(* Logix 5000 AddOnInstructionDefinition export Banner_LTF_Param_v4; software revision 33.00; part 2 of 3 *)
(* tags used below, declared in another part *)
   LTF : Banner_LTF_v4;
   Port_Data : Banner_IOL_Port_v4;
   Port : DINT;
   Local_Control : DINT;
   Command_Being_Processed : BOOL;
   Update_Archive : BOOL;
   Index_Write_Control : DINT;
   Index_Write_Inprocess : INT;
   Inprocess_Index : DINT;
(* Banner_LTF_Param_v4, continued *)

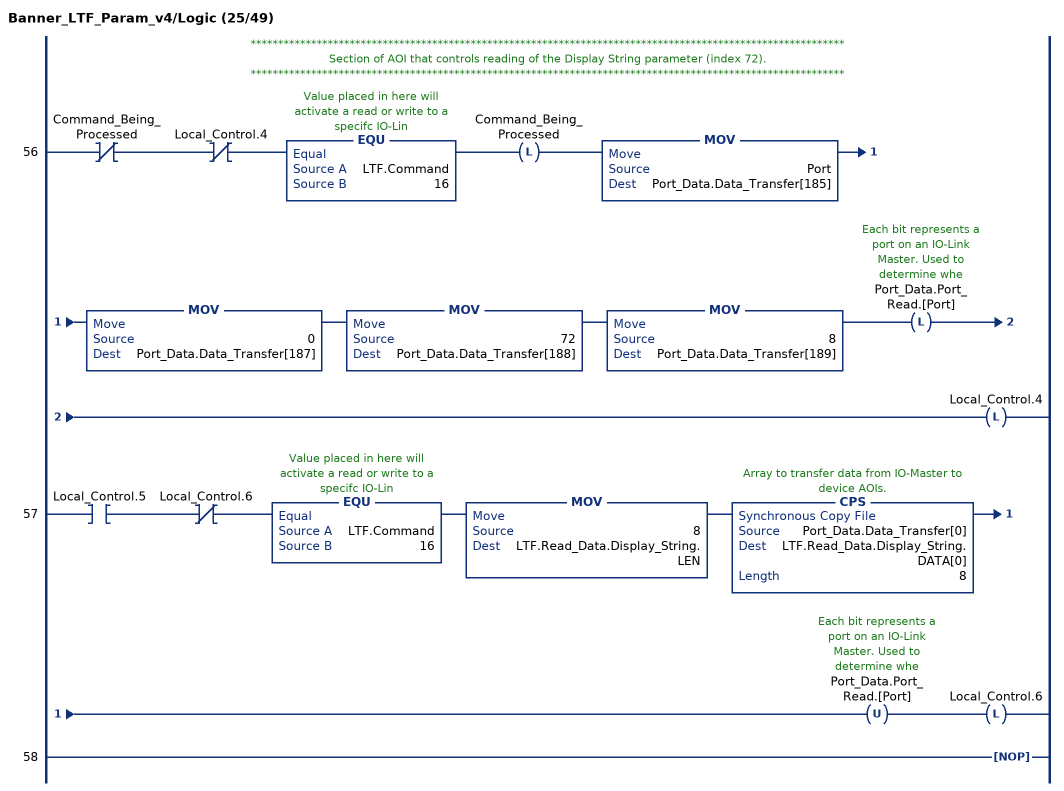
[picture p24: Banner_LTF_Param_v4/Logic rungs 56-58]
   // ************************************************************************************************************
   // Section of AOI that controls reading of the Display String parameter (index 72).
   // ************************************************************************************************************
   56: XIO(Command_Being_Processed)XIO(Local_Control.4)EQU(LTF.Command,16)OTL(Command_Being_Processed)MOV(Port,Port_Data.Data_Transfer[185])MOV(0,Port_Data.Data_Transfer[187])MOV(72,Port_Data.Data_Transfer[188])MOV(8,Port_Data.Data_Transfer[189])OTL(Port_Data.Port_Read.[Port])OTL(Local_Control.4);
   57: XIC(Local_Control.5)XIO(Local_Control.6)EQU(LTF.Command,16)MOV(8,LTF.Read_Data.Display_String.LEN)CPS(Port_Data.Data_Transfer[0],LTF.Read_Data.Display_String.DATA[0],8)OTU(Port_Data.Port_Read.[Port])OTL(Local_Control.6);
   58: NOP();
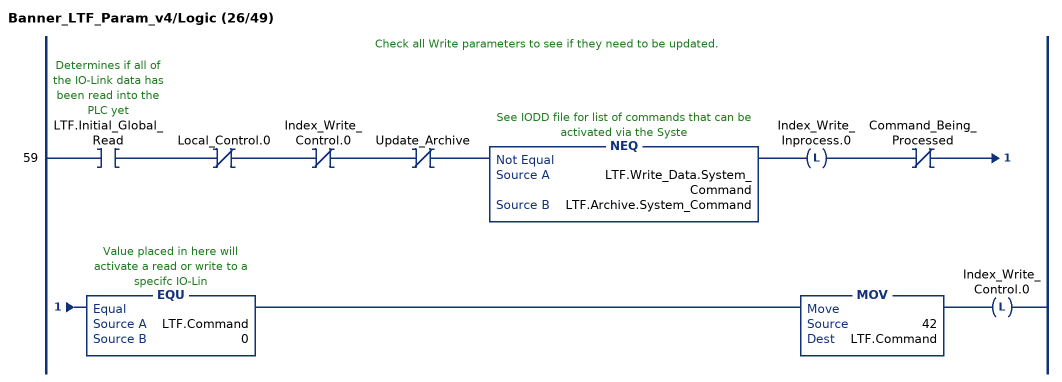
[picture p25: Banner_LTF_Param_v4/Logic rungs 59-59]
   // Check all Write parameters to see if they need to be updated.
   59: XIC(LTF.Initial_Global_Read)XIO(Local_Control.0)XIO(Index_Write_Control.0)XIO(Update_Archive)NEQ(LTF.Write_Data.System_Command,LTF.Archive.System_Command)OTL(Index_Write_Inprocess.0)XIO(Command_Being_Processed)EQU(LTF.Command,0)MOV(42,LTF.Command)OTL(Index_Write_Control.0);
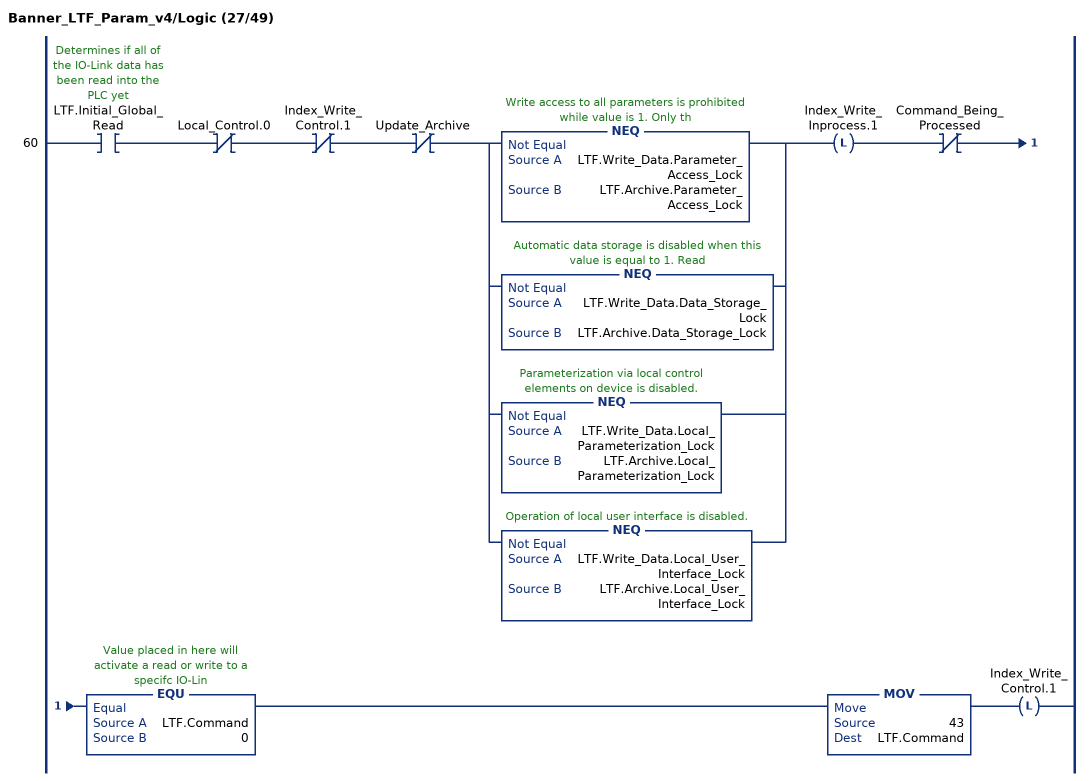
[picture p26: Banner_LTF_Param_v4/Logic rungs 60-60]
   60: XIC(LTF.Initial_Global_Read)XIO(Local_Control.0)XIO(Index_Write_Control.1)XIO(Update_Archive)[NEQ(LTF.Write_Data.Parameter_Access_Lock,LTF.Archive.Parameter_Access_Lock) ,NEQ(LTF.Write_Data.Data_Storage_Lock,LTF.Archive.Data_Storage_Lock) ,NEQ(LTF.Write_Data.Local_Parameterization_Lock,LTF.Archive.Local_Parameterization_Lock) ,NEQ(LTF.Write_Data.Local_User_Interface_Lock,LTF.Archive.Local_User_Interface_Lock) ]OTL(Index_Write_Inprocess.1)XIO(Command_Being_Processed)EQU(LTF.Command,0)MOV(43,LTF.Command)OTL(Index_Write_Control.1);
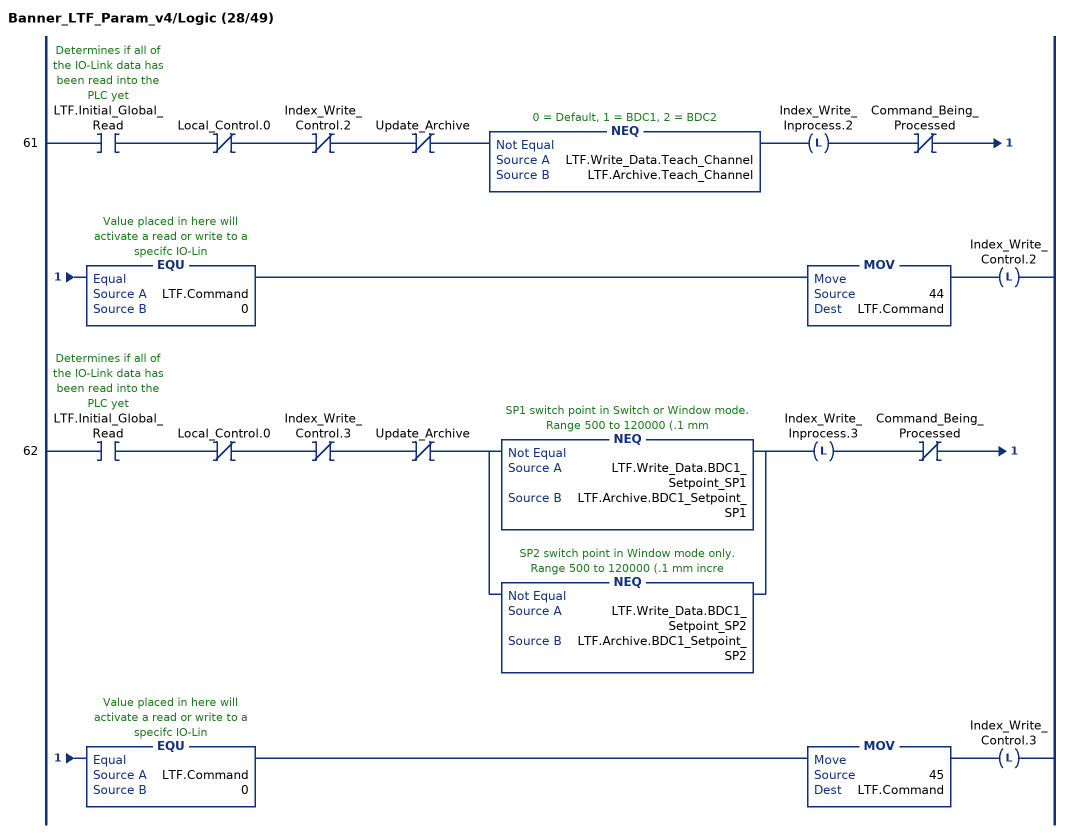
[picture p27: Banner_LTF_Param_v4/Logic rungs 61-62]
   61: XIC(LTF.Initial_Global_Read)XIO(Local_Control.0)XIO(Index_Write_Control.2)XIO(Update_Archive)NEQ(LTF.Write_Data.Teach_Channel,LTF.Archive.Teach_Channel)OTL(Index_Write_Inprocess.2)XIO(Command_Being_Processed)EQU(LTF.Command,0)MOV(44,LTF.Command)OTL(Index_Write_Control.2);
   62: XIC(LTF.Initial_Global_Read)XIO(Local_Control.0)XIO(Index_Write_Control.3)XIO(Update_Archive)[NEQ(LTF.Write_Data.BDC1_Setpoint_SP1,LTF.Archive.BDC1_Setpoint_SP1) ,NEQ(LTF.Write_Data.BDC1_Setpoint_SP2,LTF.Archive.BDC1_Setpoint_SP2) ]OTL(Index_Write_Inprocess.3)XIO(Command_Being_Processed)EQU(LTF.Command,0)MOV(45,LTF.Command)OTL(Index_Write_Control.3);
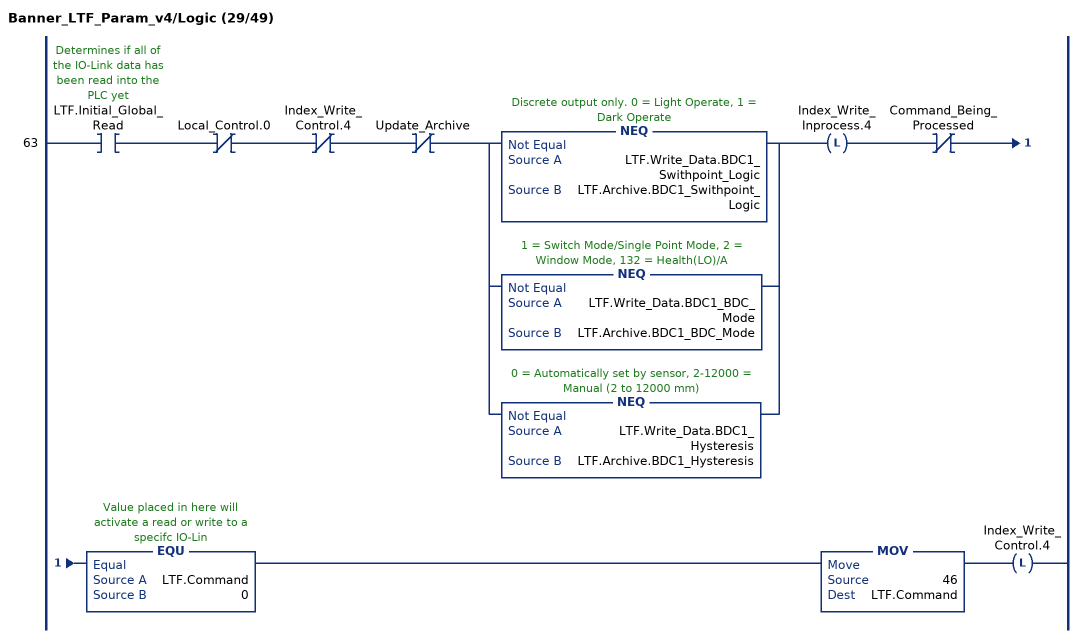
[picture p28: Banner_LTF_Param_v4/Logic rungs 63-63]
   63: XIC(LTF.Initial_Global_Read)XIO(Local_Control.0)XIO(Index_Write_Control.4)XIO(Update_Archive)[NEQ(LTF.Write_Data.BDC1_Swithpoint_Logic,LTF.Archive.BDC1_Swithpoint_Logic) ,NEQ(LTF.Write_Data.BDC1_BDC_Mode,LTF.Archive.BDC1_BDC_Mode) ,NEQ(LTF.Write_Data.BDC1_Hysteresis,LTF.Archive.BDC1_Hysteresis) ]OTL(Index_Write_Inprocess.4)XIO(Command_Being_Processed)EQU(LTF.Command,0)MOV(46,LTF.Command)OTL(Index_Write_Control.4);
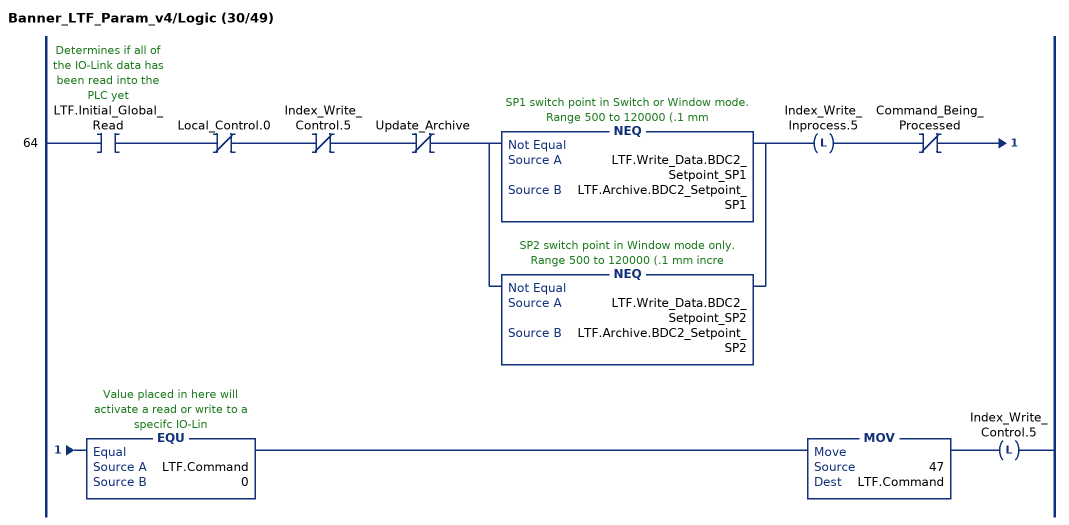
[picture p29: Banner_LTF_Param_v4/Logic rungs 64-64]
   64: XIC(LTF.Initial_Global_Read)XIO(Local_Control.0)XIO(Index_Write_Control.5)XIO(Update_Archive)[NEQ(LTF.Write_Data.BDC2_Setpoint_SP1,LTF.Archive.BDC2_Setpoint_SP1) ,NEQ(LTF.Write_Data.BDC2_Setpoint_SP2,LTF.Archive.BDC2_Setpoint_SP2) ]OTL(Index_Write_Inprocess.5)XIO(Command_Being_Processed)EQU(LTF.Command,0)MOV(47,LTF.Command)OTL(Index_Write_Control.5);
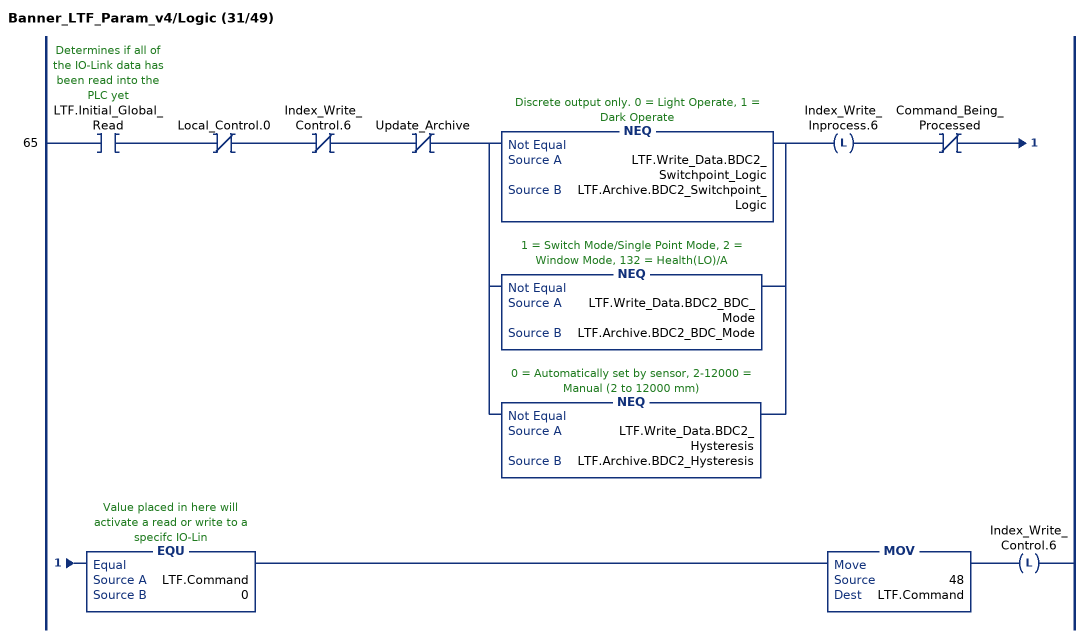
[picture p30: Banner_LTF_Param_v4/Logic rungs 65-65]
   65: XIC(LTF.Initial_Global_Read)XIO(Local_Control.0)XIO(Index_Write_Control.6)XIO(Update_Archive)[NEQ(LTF.Write_Data.BDC2_Switchpoint_Logic,LTF.Archive.BDC2_Switchpoint_Logic) ,NEQ(LTF.Write_Data.BDC2_BDC_Mode,LTF.Archive.BDC2_BDC_Mode) ,NEQ(LTF.Write_Data.BDC2_Hysteresis,LTF.Archive.BDC2_Hysteresis) ]OTL(Index_Write_Inprocess.6)XIO(Command_Being_Processed)EQU(LTF.Command,0)MOV(48,LTF.Command)OTL(Index_Write_Control.6);
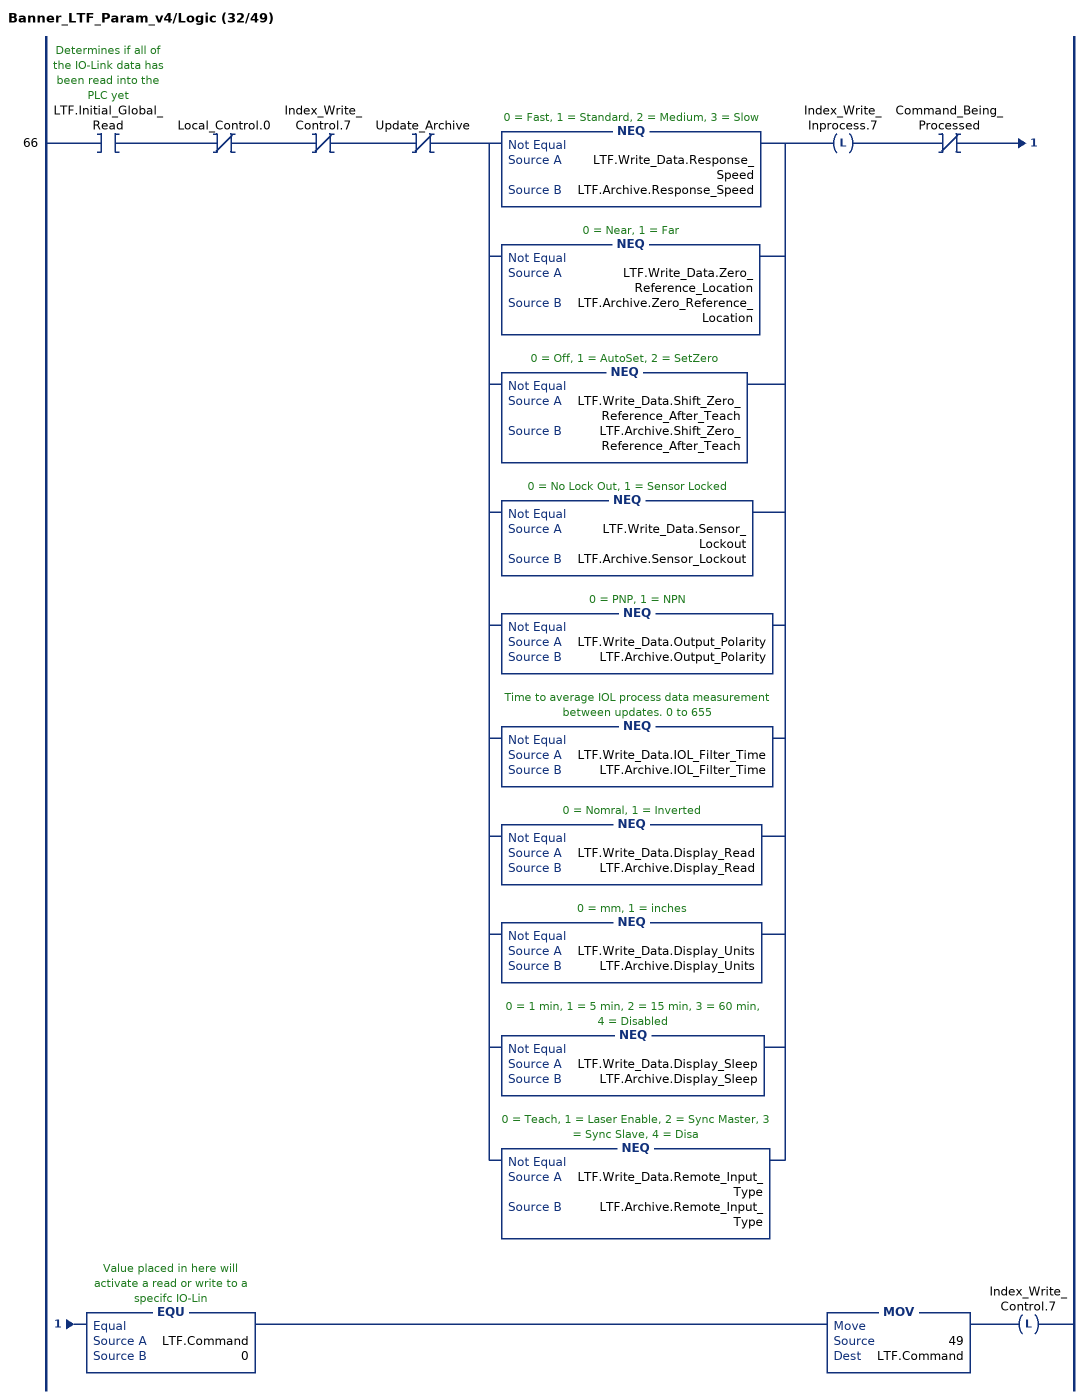
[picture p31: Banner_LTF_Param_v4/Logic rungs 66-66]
   66: XIC(LTF.Initial_Global_Read)XIO(Local_Control.0)XIO(Index_Write_Control.7)XIO(Update_Archive)[NEQ(LTF.Write_Data.Response_Speed,LTF.Archive.Response_Speed) ,NEQ(LTF.Write_Data.Zero_Reference_Location,LTF.Archive.Zero_Reference_Location) ,NEQ(LTF.Write_Data.Shift_Zero_Reference_After_Teach,LTF.Archive.Shift_Zero_Reference_After_Teach) ,NEQ(LTF.Write_Data.Sensor_Lockout,LTF.Archive.Sensor_Lockout) ,NEQ(LTF.Write_Data.Output_Polarity,LTF.Archive.Output_Polarity) ,NEQ(LTF.Write_Data.IOL_Filter_Time,LTF.Archive.IOL_Filter_Time) ,NEQ(LTF.Write_Data.Display_Read,LTF.Archive.Display_Read) ,NEQ(LTF.Write_Data.Display_Units,LTF.Archive.Display_Units) ,NEQ(LTF.Write_Data.Display_Sleep,LTF.Archive.Display_Sleep) ,NEQ(LTF.Write_Data.Remote_Input_Type,LTF.Archive.Remote_Input_Type) ]OTL(Index_Write_Inprocess.7)XIO(Command_Being_Processed)EQU(LTF.Command,0)MOV(49,LTF.Command)OTL(Index_Write_Control.7);
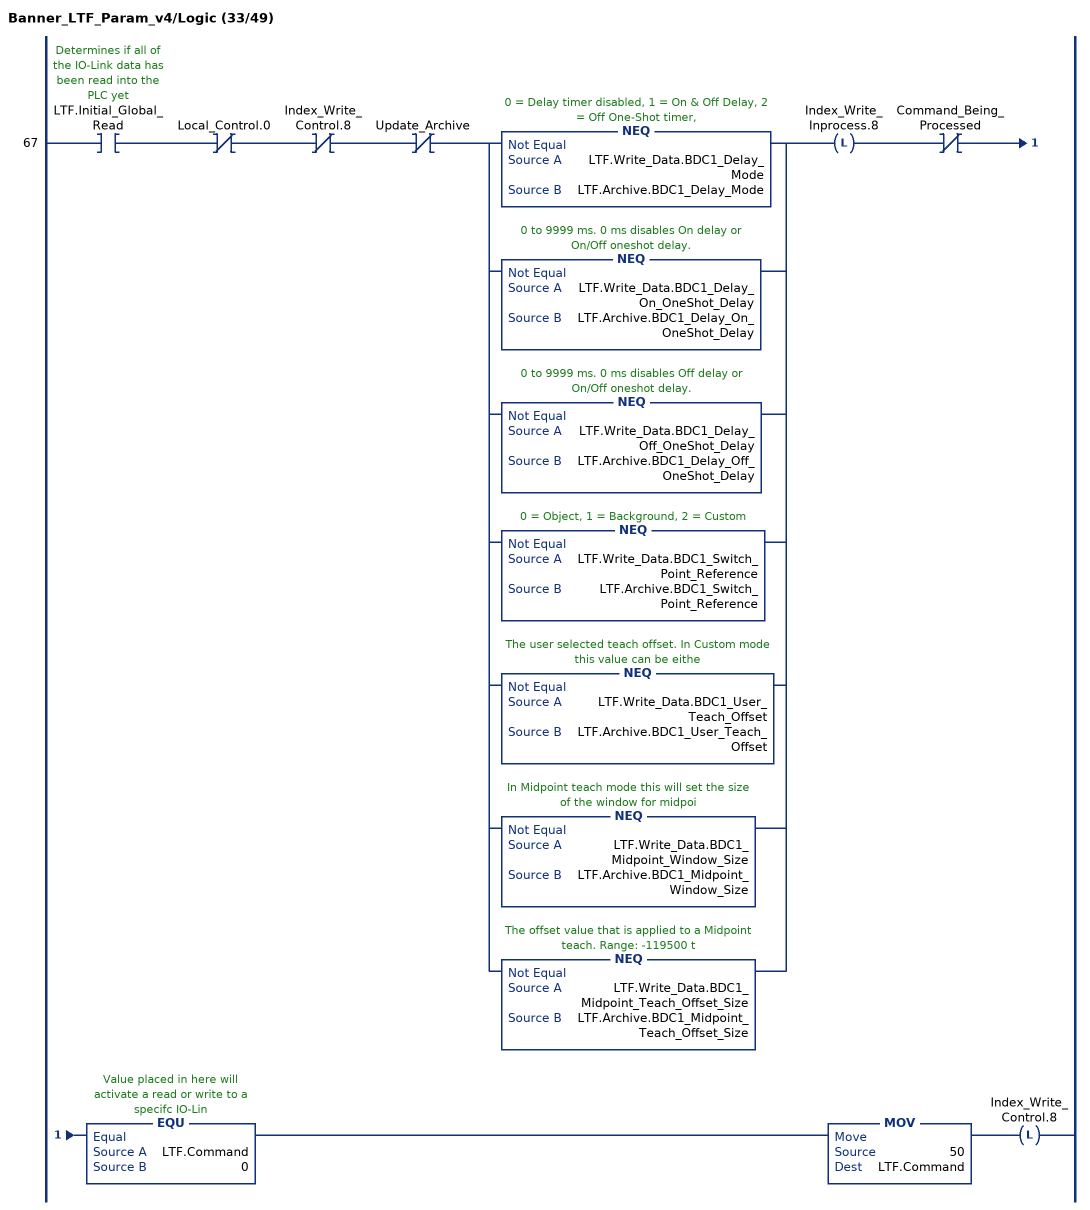
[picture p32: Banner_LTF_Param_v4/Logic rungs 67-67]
   67: XIC(LTF.Initial_Global_Read)XIO(Local_Control.0)XIO(Index_Write_Control.8)XIO(Update_Archive)[NEQ(LTF.Write_Data.BDC1_Delay_Mode,LTF.Archive.BDC1_Delay_Mode) ,NEQ(LTF.Write_Data.BDC1_Delay_On_OneShot_Delay,LTF.Archive.BDC1_Delay_On_OneShot_Delay) ,NEQ(LTF.Write_Data.BDC1_Delay_Off_OneShot_Delay,LTF.Archive.BDC1_Delay_Off_OneShot_Delay) ,NEQ(LTF.Write_Data.BDC1_Switch_Point_Reference,LTF.Archive.BDC1_Switch_Point_Reference) ,NEQ(LTF.Write_Data.BDC1_User_Teach_Offset,LTF.Archive.BDC1_User_Teach_Offset) ,NEQ(LTF.Write_Data.BDC1_Midpoint_Window_Size,LTF.Archive.BDC1_Midpoint_Window_Size) ,NEQ(LTF.Write_Data.BDC1_Midpoint_Teach_Offset_Size,LTF.Archive.BDC1_Midpoint_Teach_Offset_Size) ]OTL(Index_Write_Inprocess.8)XIO(Command_Being_Processed)EQU(LTF.Command,0)MOV(50,LTF.Command)OTL(Index_Write_Control.8);
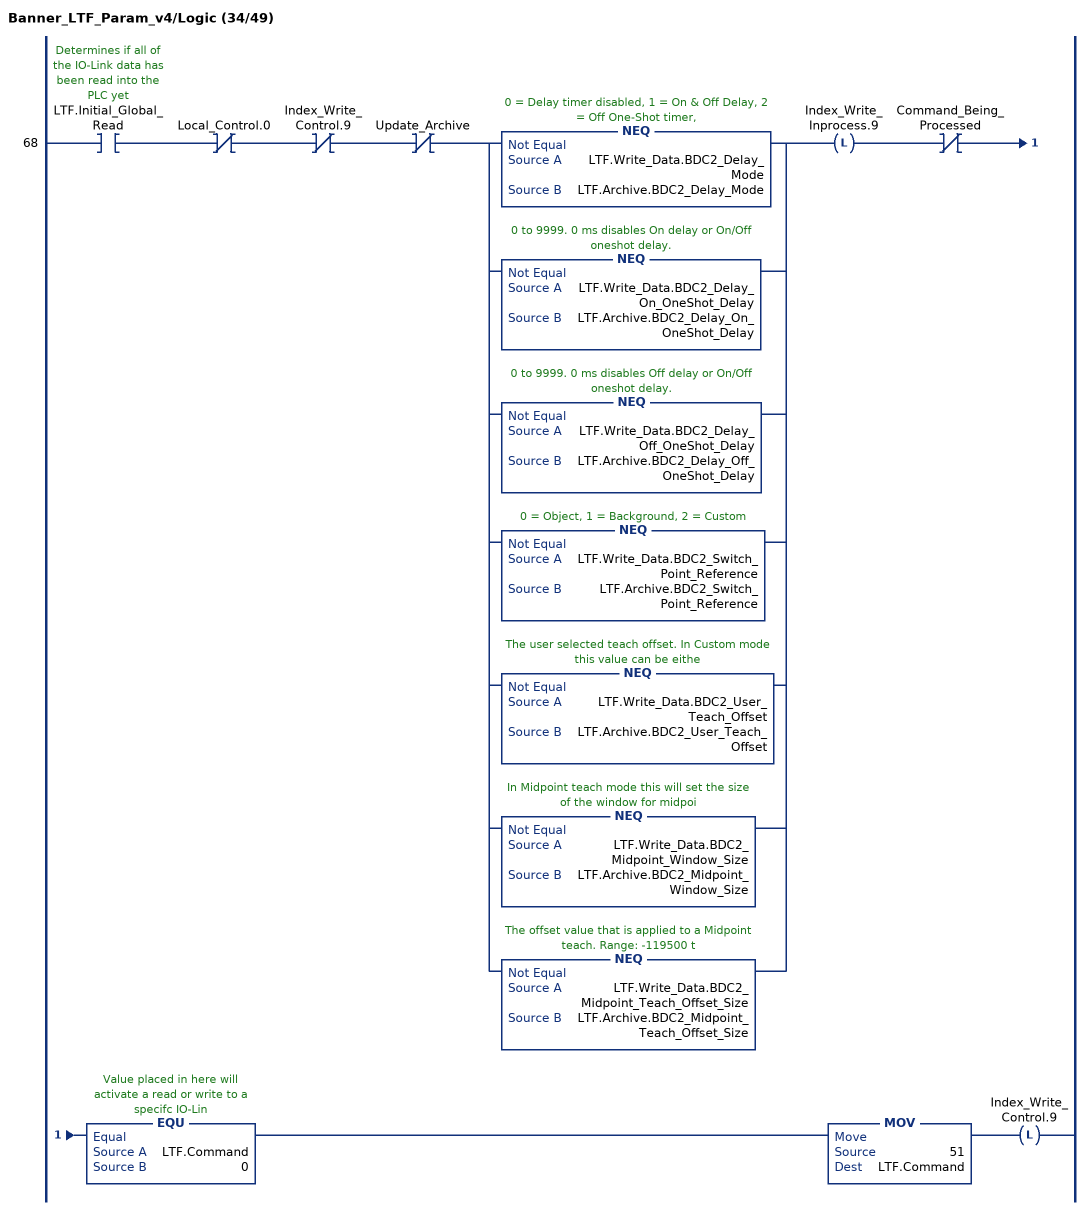
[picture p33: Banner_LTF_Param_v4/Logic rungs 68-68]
   68: XIC(LTF.Initial_Global_Read)XIO(Local_Control.0)XIO(Index_Write_Control.9)XIO(Update_Archive)[NEQ(LTF.Write_Data.BDC2_Delay_Mode,LTF.Archive.BDC2_Delay_Mode) ,NEQ(LTF.Write_Data.BDC2_Delay_On_OneShot_Delay,LTF.Archive.BDC2_Delay_On_OneShot_Delay) ,NEQ(LTF.Write_Data.BDC2_Delay_Off_OneShot_Delay,LTF.Archive.BDC2_Delay_Off_OneShot_Delay) ,NEQ(LTF.Write_Data.BDC2_Switch_Point_Reference,LTF.Archive.BDC2_Switch_Point_Reference) ,NEQ(LTF.Write_Data.BDC2_User_Teach_Offset,LTF.Archive.BDC2_User_Teach_Offset) ,NEQ(LTF.Write_Data.BDC2_Midpoint_Window_Size,LTF.Archive.BDC2_Midpoint_Window_Size) ,NEQ(LTF.Write_Data.BDC2_Midpoint_Teach_Offset_Size,LTF.Archive.BDC2_Midpoint_Teach_Offset_Size) ]OTL(Index_Write_Inprocess.9)XIO(Command_Being_Processed)EQU(LTF.Command,0)MOV(51,LTF.Command)OTL(Index_Write_Control.9);
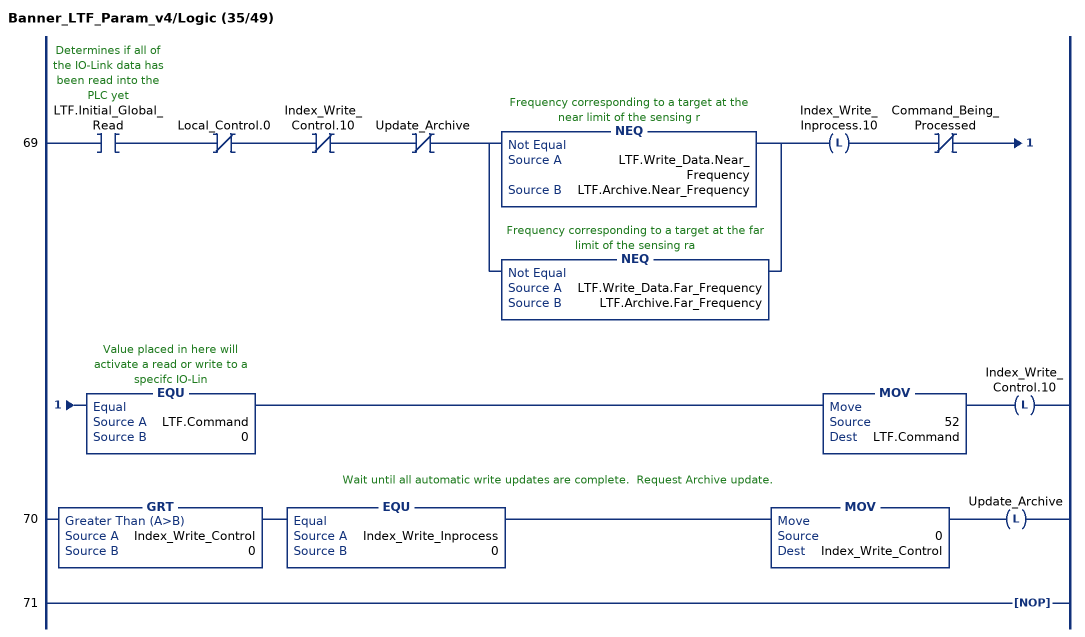
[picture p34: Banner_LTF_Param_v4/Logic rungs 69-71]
   69: XIC(LTF.Initial_Global_Read)XIO(Local_Control.0)XIO(Index_Write_Control.10)XIO(Update_Archive)[NEQ(LTF.Write_Data.Near_Frequency,LTF.Archive.Near_Frequency) ,NEQ(LTF.Write_Data.Far_Frequency,LTF.Archive.Far_Frequency) ]OTL(Index_Write_Inprocess.10)XIO(Command_Being_Processed)EQU(LTF.Command,0)MOV(52,LTF.Command)OTL(Index_Write_Control.10);
   // Wait until all automatic write updates are complete.  Request Archive update.
   70: GRT(Index_Write_Control,0)EQU(Index_Write_Inprocess,0)MOV(0,Index_Write_Control)OTL(Update_Archive);
   71: NOP();
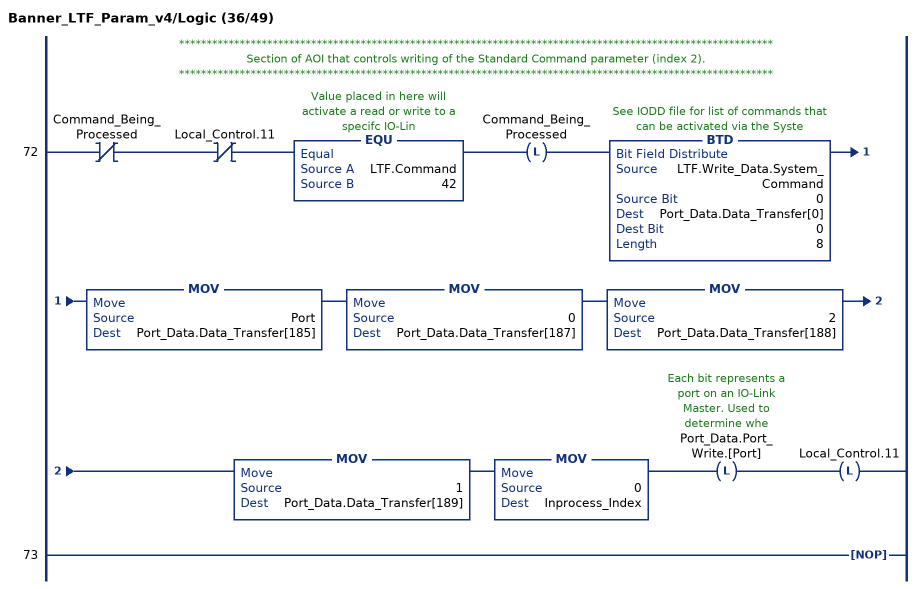
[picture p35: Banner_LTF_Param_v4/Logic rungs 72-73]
   // ************************************************************************************************************
   // Section of AOI that controls writing of the Standard Command parameter (index 2).
   // ************************************************************************************************************
   72: XIO(Command_Being_Processed)XIO(Local_Control.11)EQU(LTF.Command,42)OTL(Command_Being_Processed)BTD(LTF.Write_Data.System_Command,0,Port_Data.Data_Transfer[0],0,8)MOV(Port,Port_Data.Data_Transfer[185])MOV(0,Port_Data.Data_Transfer[187])MOV(2,Port_Data.Data_Transfer[188])MOV(1,Port_Data.Data_Transfer[189])MOV(0,Inprocess_Index)OTL(Port_Data.Port_Write.[Port])OTL(Local_Control.11);
   73: NOP();
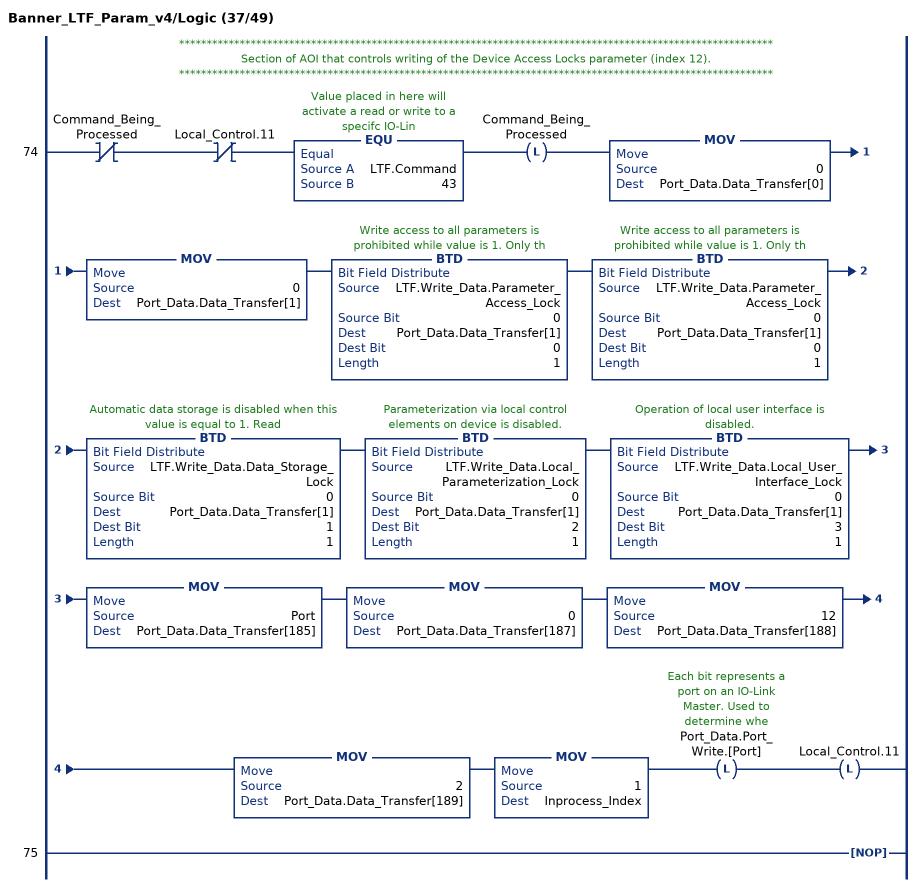
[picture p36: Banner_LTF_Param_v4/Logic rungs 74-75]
   // ************************************************************************************************************
   // Section of AOI that controls writing of the Device Access Locks parameter (index 12).
   // ************************************************************************************************************
   74: XIO(Command_Being_Processed)XIO(Local_Control.11)EQU(LTF.Command,43)OTL(Command_Being_Processed)MOV(0,Port_Data.Data_Transfer[0])MOV(0,Port_Data.Data_Transfer[1])BTD(LTF.Write_Data.Parameter_Access_Lock,0,Port_Data.Data_Transfer[1],0,1)BTD(LTF.Write_Data.Parameter_Access_Lock,0,Port_Data.Data_Transfer[1],0,1)BTD(LTF.Write_Data.Data_Storage_Lock,0,Port_Data.Data_Transfer[1],1,1)BTD(LTF.Write_Data.Local_Parameterization_Lock,0,Port_Data.Data_Transfer[1],2,1)BTD(LTF.Write_Data.Local_User_Interface_Lock,0,Port_Data.Data_Transfer[1],3,1)MOV(Port,Port_Data.Data_Transfer[185])MOV(0,Port_Data.Data_Transfer[187])MOV(12,Port_Data.Data_Transfer[188])MOV(2,Port_Data.Data_Transfer[189])MOV(1,Inprocess_Index)OTL(Port_Data.Port_Write.[Port])OTL(Local_Control.11);
   75: NOP();
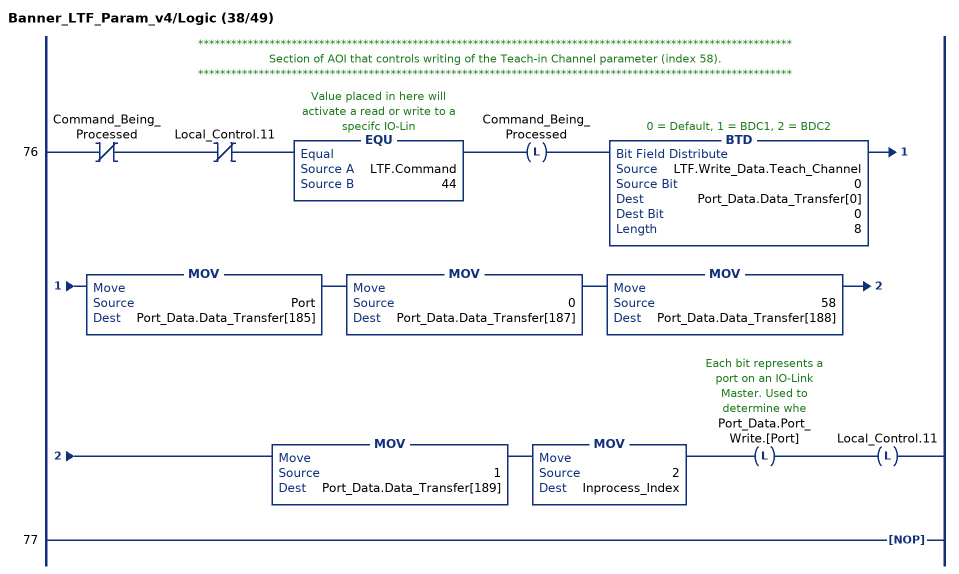
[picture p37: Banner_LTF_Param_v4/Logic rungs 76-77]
   // ************************************************************************************************************
   // Section of AOI that controls writing of the Teach-in Channel parameter (index 58).
   // ************************************************************************************************************
   76: XIO(Command_Being_Processed)XIO(Local_Control.11)EQU(LTF.Command,44)OTL(Command_Being_Processed)BTD(LTF.Write_Data.Teach_Channel,0,Port_Data.Data_Transfer[0],0,8)MOV(Port,Port_Data.Data_Transfer[185])MOV(0,Port_Data.Data_Transfer[187])MOV(58,Port_Data.Data_Transfer[188])MOV(1,Port_Data.Data_Transfer[189])MOV(2,Inprocess_Index)OTL(Port_Data.Port_Write.[Port])OTL(Local_Control.11);
   77: NOP();
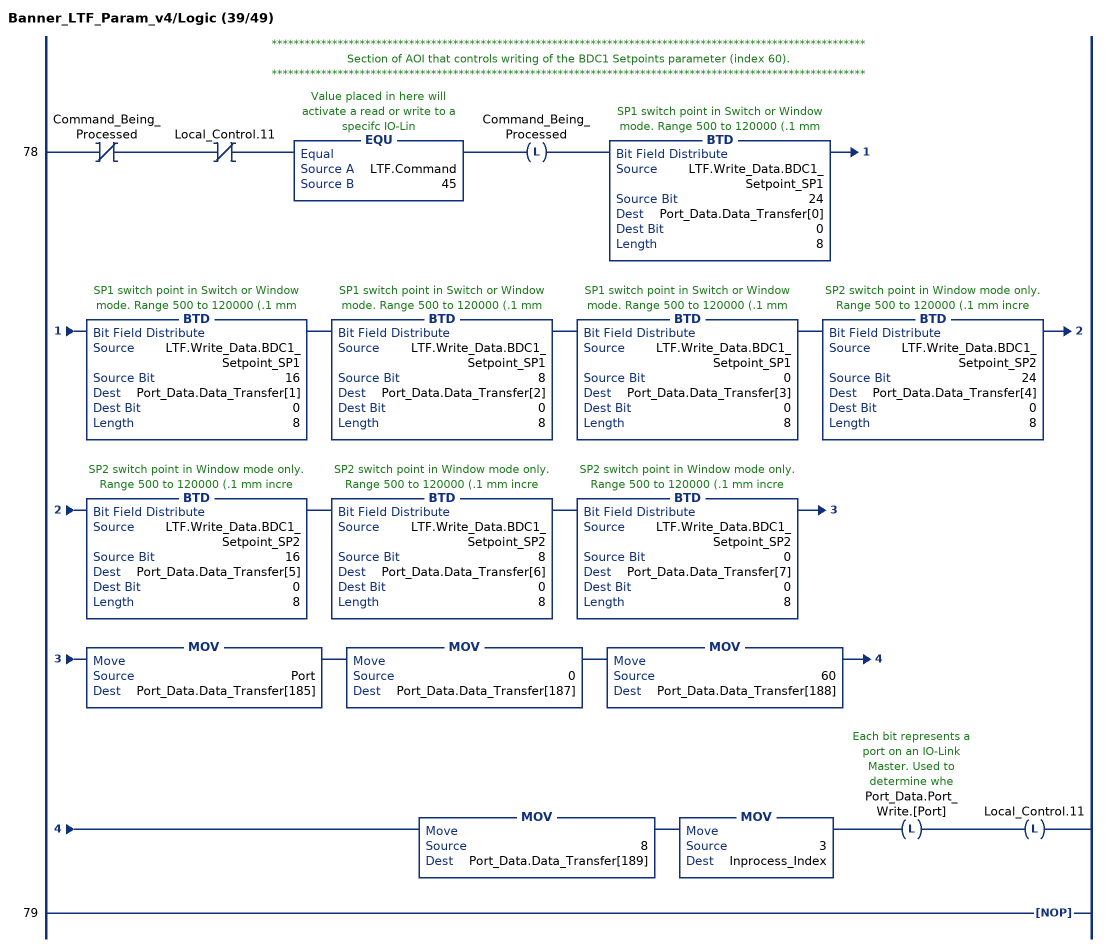
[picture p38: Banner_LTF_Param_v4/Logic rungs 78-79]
   // ************************************************************************************************************
   // Section of AOI that controls writing of the BDC1 Setpoints parameter (index 60).
   // ************************************************************************************************************
   78: XIO(Command_Being_Processed)XIO(Local_Control.11)EQU(LTF.Command,45)OTL(Command_Being_Processed)BTD(LTF.Write_Data.BDC1_Setpoint_SP1,24,Port_Data.Data_Transfer[0],0,8)BTD(LTF.Write_Data.BDC1_Setpoint_SP1,16,Port_Data.Data_Transfer[1],0,8)BTD(LTF.Write_Data.BDC1_Setpoint_SP1,8,Port_Data.Data_Transfer[2],0,8)BTD(LTF.Write_Data.BDC1_Setpoint_SP1,0,Port_Data.Data_Transfer[3],0,8)BTD(LTF.Write_Data.BDC1_Setpoint_SP2,24,Port_Data.Data_Transfer[4],0,8)BTD(LTF.Write_Data.BDC1_Setpoint_SP2,16,Port_Data.Data_Transfer[5],0,8)BTD(LTF.Write_Data.BDC1_Setpoint_SP2,8,Port_Data.Data_Transfer[6],0,8)BTD(LTF.Write_Data.BDC1_Setpoint_SP2,0,Port_Data.Data_Transfer[7],0,8)MOV(Port,Port_Data.Data_Transfer[185])MOV(0,Port_Data.Data_Transfer[187])MOV(60,Port_Data.Data_Transfer[188])MOV(8,Port_Data.Data_Transfer[189])MOV(3,Inprocess_Index)OTL(Port_Data.Port_Write.[Port])OTL(Local_Control.11);
   79: NOP();
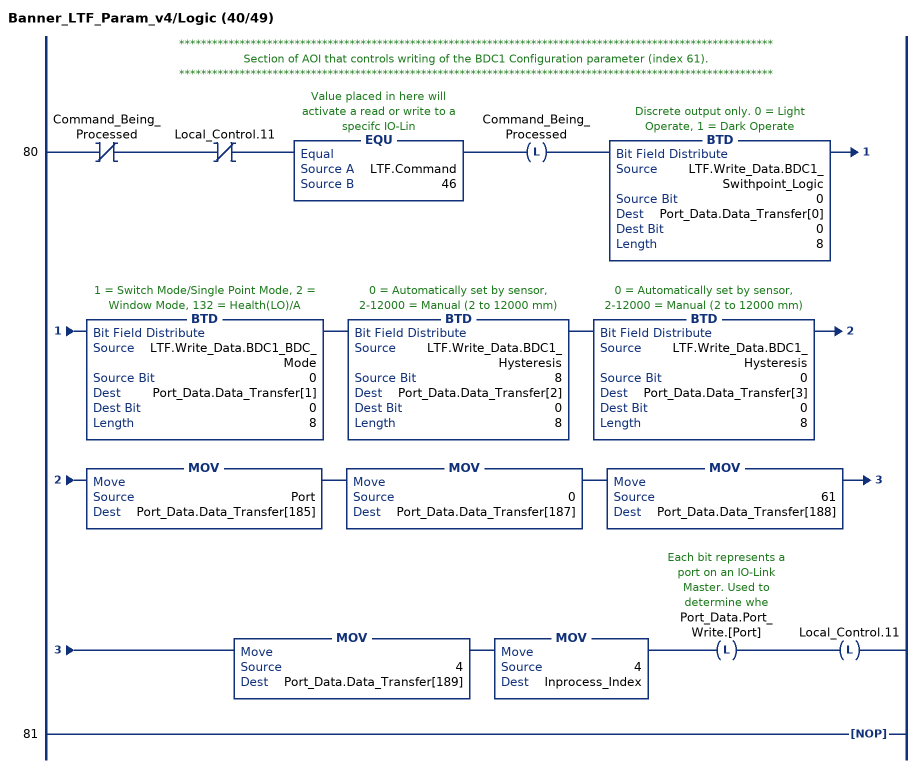
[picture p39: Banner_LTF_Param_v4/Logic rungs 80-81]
   // ************************************************************************************************************
   // Section of AOI that controls writing of the BDC1 Configuration parameter (index 61).
   // ************************************************************************************************************
   80: XIO(Command_Being_Processed)XIO(Local_Control.11)EQU(LTF.Command,46)OTL(Command_Being_Processed)BTD(LTF.Write_Data.BDC1_Swithpoint_Logic,0,Port_Data.Data_Transfer[0],0,8)BTD(LTF.Write_Data.BDC1_BDC_Mode,0,Port_Data.Data_Transfer[1],0,8)BTD(LTF.Write_Data.BDC1_Hysteresis,8,Port_Data.Data_Transfer[2],0,8)BTD(LTF.Write_Data.BDC1_Hysteresis,0,Port_Data.Data_Transfer[3],0,8)MOV(Port,Port_Data.Data_Transfer[185])MOV(0,Port_Data.Data_Transfer[187])MOV(61,Port_Data.Data_Transfer[188])MOV(4,Port_Data.Data_Transfer[189])MOV(4,Inprocess_Index)OTL(Port_Data.Port_Write.[Port])OTL(Local_Control.11);
   81: NOP();
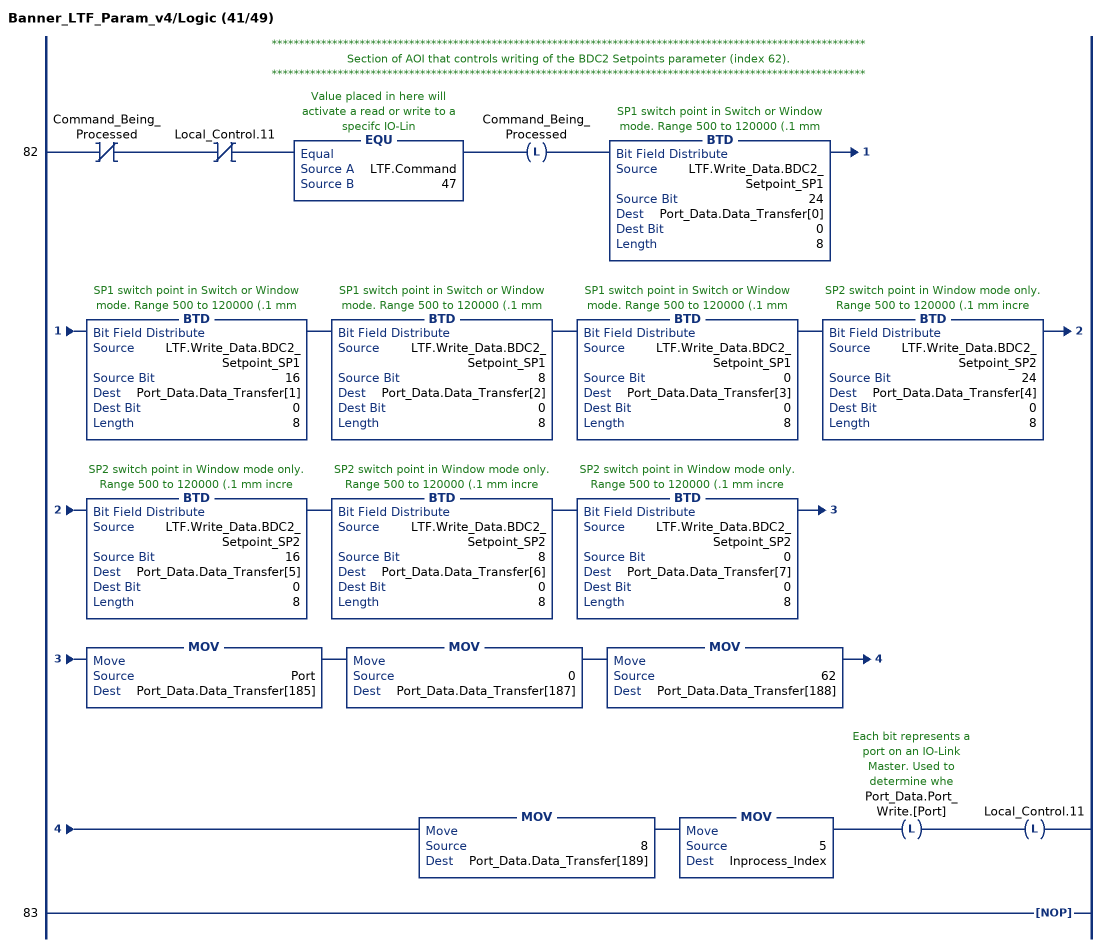
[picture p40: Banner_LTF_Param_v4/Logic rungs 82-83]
   // ************************************************************************************************************
   // Section of AOI that controls writing of the BDC2 Setpoints parameter (index 62).
   // ************************************************************************************************************
   82: XIO(Command_Being_Processed)XIO(Local_Control.11)EQU(LTF.Command,47)OTL(Command_Being_Processed)BTD(LTF.Write_Data.BDC2_Setpoint_SP1,24,Port_Data.Data_Transfer[0],0,8)BTD(LTF.Write_Data.BDC2_Setpoint_SP1,16,Port_Data.Data_Transfer[1],0,8)BTD(LTF.Write_Data.BDC2_Setpoint_SP1,8,Port_Data.Data_Transfer[2],0,8)BTD(LTF.Write_Data.BDC2_Setpoint_SP1,0,Port_Data.Data_Transfer[3],0,8)BTD(LTF.Write_Data.BDC2_Setpoint_SP2,24,Port_Data.Data_Transfer[4],0,8)BTD(LTF.Write_Data.BDC2_Setpoint_SP2,16,Port_Data.Data_Transfer[5],0,8)BTD(LTF.Write_Data.BDC2_Setpoint_SP2,8,Port_Data.Data_Transfer[6],0,8)BTD(LTF.Write_Data.BDC2_Setpoint_SP2,0,Port_Data.Data_Transfer[7],0,8)MOV(Port,Port_Data.Data_Transfer[185])MOV(0,Port_Data.Data_Transfer[187])MOV(62,Port_Data.Data_Transfer[188])MOV(8,Port_Data.Data_Transfer[189])MOV(5,Inprocess_Index)OTL(Port_Data.Port_Write.[Port])OTL(Local_Control.11);
   83: NOP();
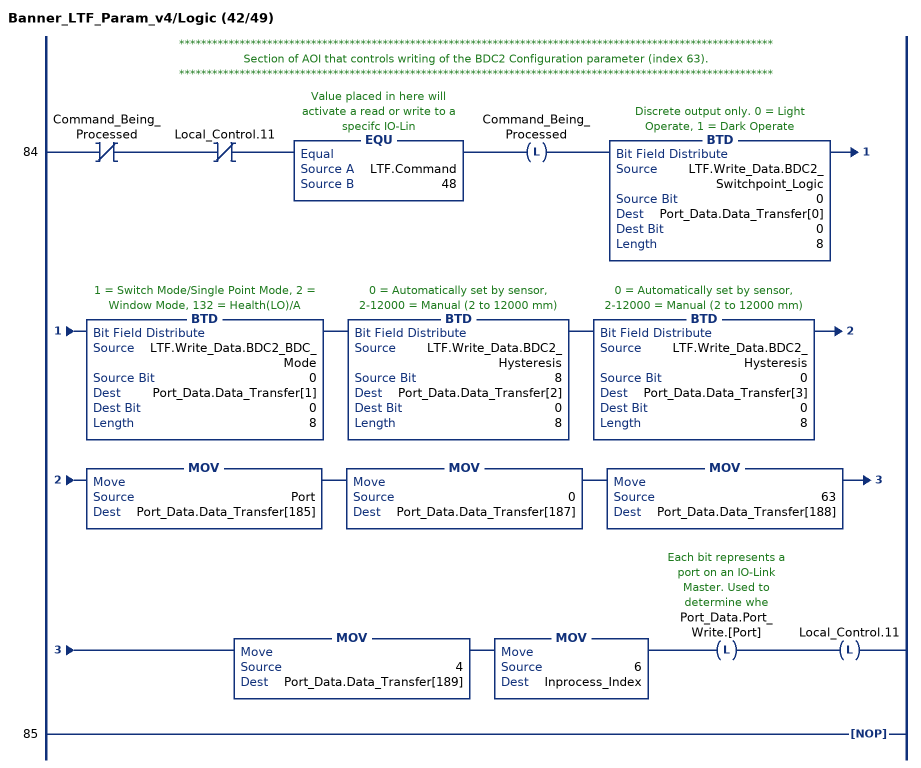
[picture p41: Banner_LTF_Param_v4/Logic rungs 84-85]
   // ************************************************************************************************************
   // Section of AOI that controls writing of the BDC2 Configuration parameter (index 63).
   // ************************************************************************************************************
   84: XIO(Command_Being_Processed)XIO(Local_Control.11)EQU(LTF.Command,48)OTL(Command_Being_Processed)BTD(LTF.Write_Data.BDC2_Switchpoint_Logic,0,Port_Data.Data_Transfer[0],0,8)BTD(LTF.Write_Data.BDC2_BDC_Mode,0,Port_Data.Data_Transfer[1],0,8)BTD(LTF.Write_Data.BDC2_Hysteresis,8,Port_Data.Data_Transfer[2],0,8)BTD(LTF.Write_Data.BDC2_Hysteresis,0,Port_Data.Data_Transfer[3],0,8)MOV(Port,Port_Data.Data_Transfer[185])MOV(0,Port_Data.Data_Transfer[187])MOV(63,Port_Data.Data_Transfer[188])MOV(4,Port_Data.Data_Transfer[189])MOV(6,Inprocess_Index)OTL(Port_Data.Port_Write.[Port])OTL(Local_Control.11);
   85: NOP();
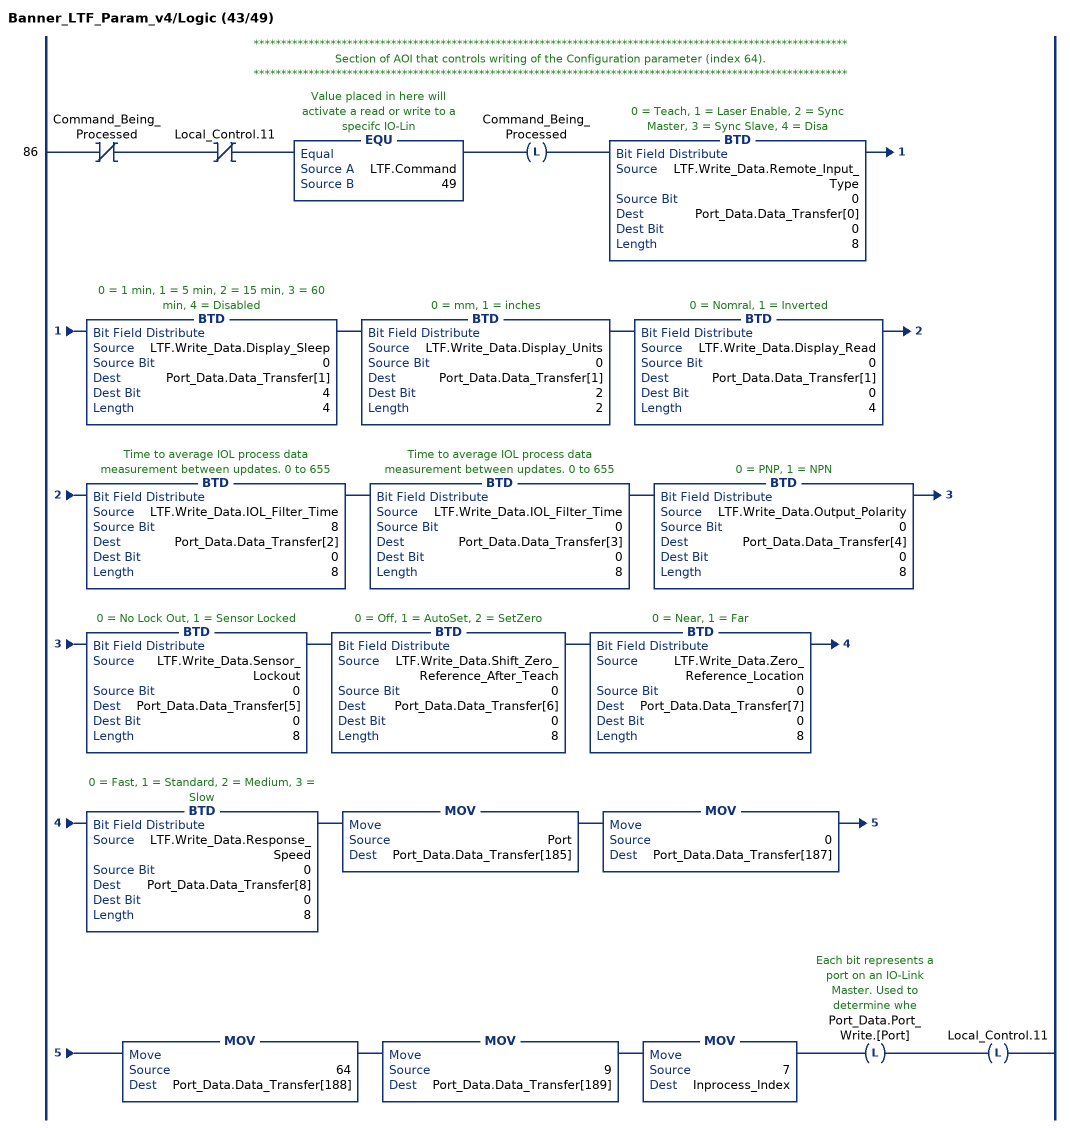
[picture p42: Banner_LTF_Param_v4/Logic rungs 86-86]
   // ************************************************************************************************************
   // Section of AOI that controls writing of the Configuration parameter (index 64).
   // ************************************************************************************************************
   86: XIO(Command_Being_Processed)XIO(Local_Control.11)EQU(LTF.Command,49)OTL(Command_Being_Processed)BTD(LTF.Write_Data.Remote_Input_Type,0,Port_Data.Data_Transfer[0],0,8)BTD(LTF.Write_Data.Display_Sleep,0,Port_Data.Data_Transfer[1],4,4)BTD(LTF.Write_Data.Display_Units,0,Port_Data.Data_Transfer[1],2,2)BTD(LTF.Write_Data.Display_Read,0,Port_Data.Data_Transfer[1],0,4)BTD(LTF.Write_Data.IOL_Filter_Time,8,Port_Data.Data_Transfer[2],0,8)BTD(LTF.Write_Data.IOL_Filter_Time,0,Port_Data.Data_Transfer[3],0,8)BTD(LTF.Write_Data.Output_Polarity,0,Port_Data.Data_Transfer[4],0,8)BTD(LTF.Write_Data.Sensor_Lockout,0,Port_Data.Data_Transfer[5],0,8)BTD(LTF.Write_Data.Shift_Zero_Reference_After_Teach,0,Port_Data.Data_Transfer[6],0,8)BTD(LTF.Write_Data.Zero_Reference_Location,0,Port_Data.Data_Transfer[7],0,8)BTD(LTF.Write_Data.Response_Speed,0,Port_Data.Data_Transfer[8],0,8)MOV(Port,Port_Data.Data_Transfer[185])MOV(0,Port_Data.Data_Transfer[187])MOV(64,Port_Data.Data_Transfer[188])MOV(9,Port_Data.Data_Transfer[189])MOV(7,Inprocess_Index)OTL(Port_Data.Port_Write.[Port])OTL(Local_Control.11);
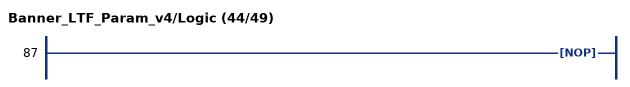
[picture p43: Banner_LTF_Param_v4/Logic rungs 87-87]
   87: NOP();
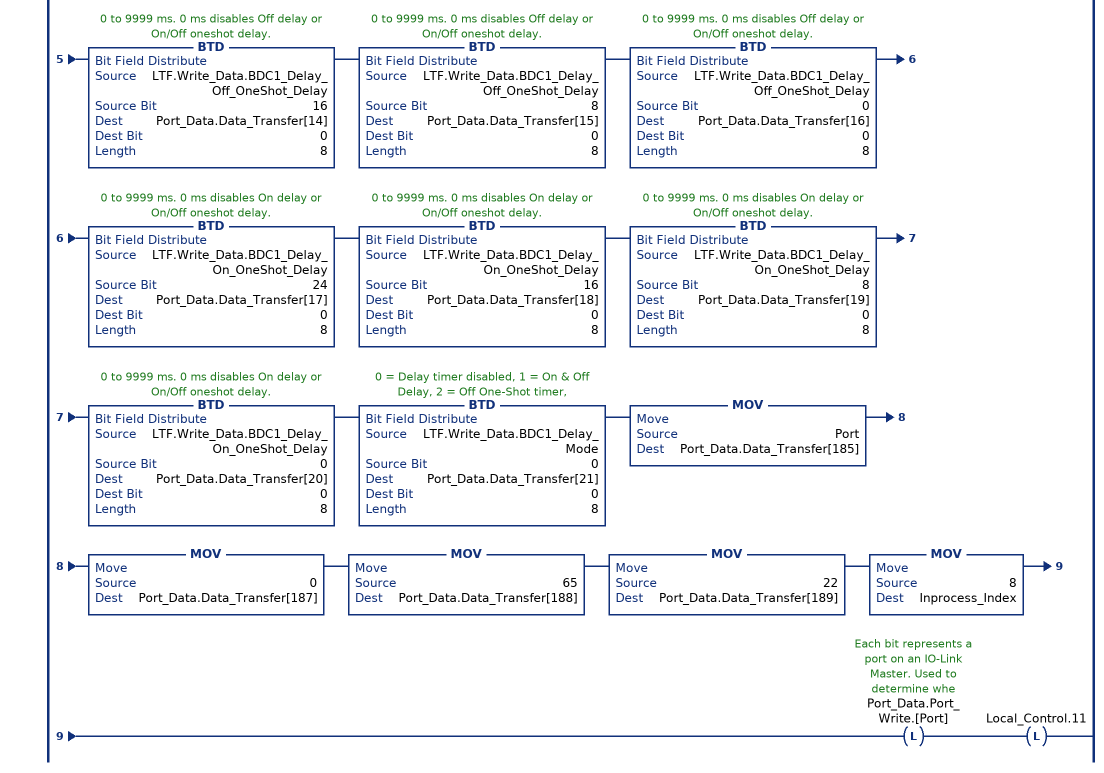
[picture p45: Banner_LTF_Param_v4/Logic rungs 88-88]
   // ************************************************************************************************************
   // Section of AOI that controls writing of the BDC1 Vendor Specific Configuration parameter (index 65).
   // ************************************************************************************************************
   88: XIO(Command_Being_Processed)XIO(Local_Control.11)EQU(LTF.Command,50)OTL(Command_Being_Processed)BTD(LTF.Write_Data.BDC1_Midpoint_Teach_Offset_Size,24,Port_Data.Data_Transfer[0],0,8)BTD(LTF.Write_Data.BDC1_Midpoint_Teach_Offset_Size,16,Port_Data.Data_Transfer[1],0,8)BTD(LTF.Write_Data.BDC1_Midpoint_Teach_Offset_Size,8,Port_Data.Data_Transfer[2],0,8)BTD(LTF.Write_Data.BDC1_Midpoint_Teach_Offset_Size,0,Port_Data.Data_Transfer[3],0,8)BTD(LTF.Write_Data.BDC1_Midpoint_Window_Size,24,Port_Data.Data_Transfer[4],0,8)BTD(LTF.Write_Data.BDC1_Midpoint_Window_Size,16,Port_Data.Data_Transfer[5],0,8)BTD(LTF.Write_Data.BDC1_Midpoint_Window_Size,8,Port_Data.Data_Transfer[6],0,8)BTD(LTF.Write_Data.BDC1_Midpoint_Window_Size,0,Port_Data.Data_Transfer[7],0,8)BTD(LTF.Write_Data.BDC1_User_Teach_Offset,24,Port_Data.Data_Transfer[8],0,8)BTD(LTF.Write_Data.BDC1_User_Teach_Offset,16,Port_Data.Data_Transfer[9],0,8)BTD(LTF.Write_Data.BDC1_User_Teach_Offset,8,Port_Data.Data_Transfer[10],0,8)BTD(LTF.Write_Data.BDC1_User_Teach_Offset,0,Port_Data.Data_Transfer[11],0,8)BTD(LTF.Write_Data.BDC1_Switch_Point_Reference,0,Port_Data.Data_Transfer[12],0,8)BTD(LTF.Write_Data.BDC1_Delay_Off_OneShot_Delay,24,Port_Data.Data_Transfer[13],0,8)BTD(LTF.Write_Data.BDC1_Delay_Off_OneShot_Delay,16,Port_Data.Data_Transfer[14],0,8)BTD(LTF.Write_Data.BDC1_Delay_Off_OneShot_Delay,8,Port_Data.Data_Transfer[15],0,8)BTD(LTF.Write_Data.BDC1_Delay_Off_OneShot_Delay,0,Port_Data.Data_Transfer[16],0,8)BTD(LTF.Write_Data.BDC1_Delay_On_OneShot_Delay,24,Port_Data.Data_Transfer[17],0,8)BTD(LTF.Write_Data.BDC1_Delay_On_OneShot_Delay,16,Port_Data.Data_Transfer[18],0,8)BTD(LTF.Write_Data.BDC1_Delay_On_OneShot_Delay,8,Port_Data.Data_Transfer[19],0,8)BTD(LTF.Write_Data.BDC1_Delay_On_OneShot_Delay,0,Port_Data.Data_Transfer[20],0,8)BTD(LTF.Write_Data.BDC1_Delay_Mode,0,Port_Data.Data_Transfer[21],0,8)MOV(Port,Port_Data.Data_Transfer[185])MOV(0,Port_Data.Data_Transfer[187])MOV(65,Port_Data.Data_Transfer[188])MOV(22,Port_Data.Data_Transfer[189])MOV(8,Inprocess_Index)OTL(Port_Data.Port_Write.[Port])OTL(Local_Control.11);
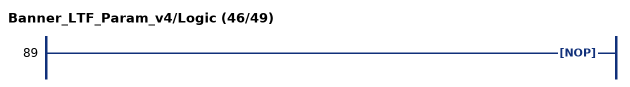
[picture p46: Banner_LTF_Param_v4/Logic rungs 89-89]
   89: NOP();
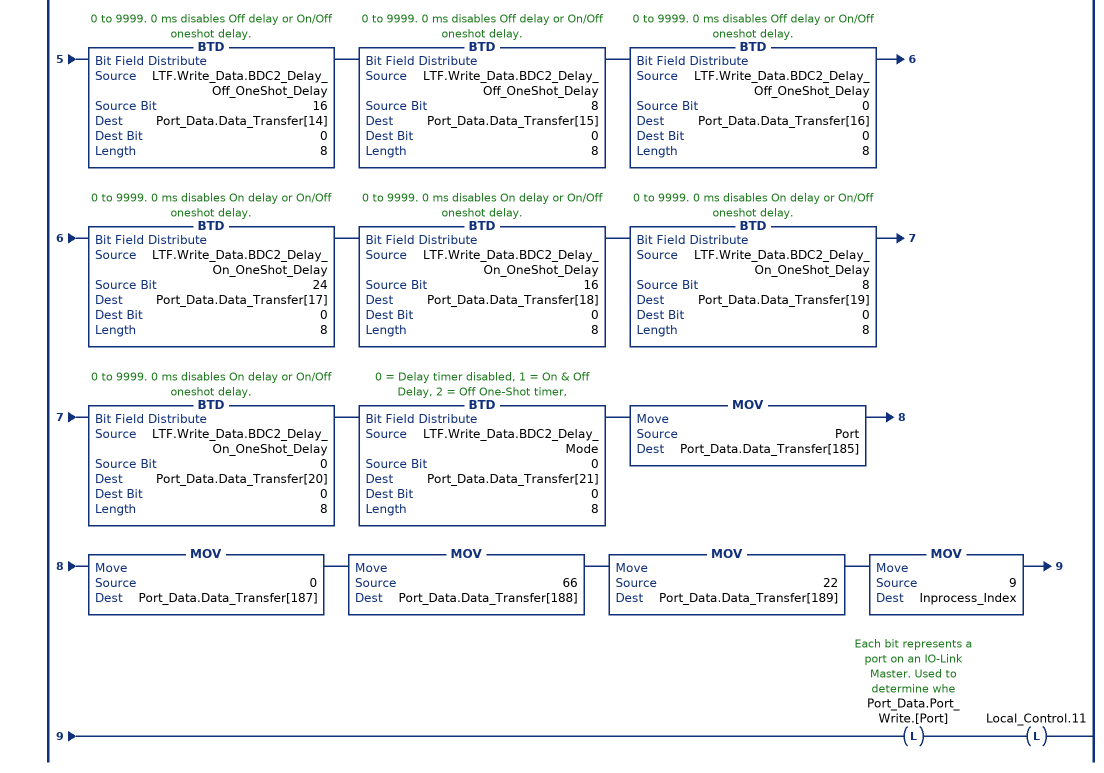
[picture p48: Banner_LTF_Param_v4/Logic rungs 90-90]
   // ************************************************************************************************************
   // Section of AOI that controls writing of the BDC2 Vendor Specific Configuration parameter (index 66).
   // ************************************************************************************************************
   90: XIO(Command_Being_Processed)XIO(Local_Control.11)EQU(LTF.Command,51)OTL(Command_Being_Processed)BTD(LTF.Write_Data.BDC2_Midpoint_Teach_Offset_Size,24,Port_Data.Data_Transfer[0],0,8)BTD(LTF.Write_Data.BDC2_Midpoint_Teach_Offset_Size,16,Port_Data.Data_Transfer[1],0,8)BTD(LTF.Write_Data.BDC2_Midpoint_Teach_Offset_Size,8,Port_Data.Data_Transfer[2],0,8)BTD(LTF.Write_Data.BDC2_Midpoint_Teach_Offset_Size,0,Port_Data.Data_Transfer[3],0,8)BTD(LTF.Write_Data.BDC2_Midpoint_Window_Size,24,Port_Data.Data_Transfer[4],0,8)BTD(LTF.Write_Data.BDC2_Midpoint_Window_Size,16,Port_Data.Data_Transfer[5],0,8)BTD(LTF.Write_Data.BDC2_Midpoint_Window_Size,8,Port_Data.Data_Transfer[6],0,8)BTD(LTF.Write_Data.BDC2_Midpoint_Window_Size,0,Port_Data.Data_Transfer[7],0,8)BTD(LTF.Write_Data.BDC2_User_Teach_Offset,24,Port_Data.Data_Transfer[8],0,8)BTD(LTF.Write_Data.BDC2_User_Teach_Offset,16,Port_Data.Data_Transfer[9],0,8)BTD(LTF.Write_Data.BDC2_User_Teach_Offset,8,Port_Data.Data_Transfer[10],0,8)BTD(LTF.Write_Data.BDC2_User_Teach_Offset,0,Port_Data.Data_Transfer[11],0,8)BTD(LTF.Write_Data.BDC2_Switch_Point_Reference,0,Port_Data.Data_Transfer[12],0,8)BTD(LTF.Write_Data.BDC2_Delay_Off_OneShot_Delay,24,Port_Data.Data_Transfer[13],0,8)BTD(LTF.Write_Data.BDC2_Delay_Off_OneShot_Delay,16,Port_Data.Data_Transfer[14],0,8)BTD(LTF.Write_Data.BDC2_Delay_Off_OneShot_Delay,8,Port_Data.Data_Transfer[15],0,8)BTD(LTF.Write_Data.BDC2_Delay_Off_OneShot_Delay,0,Port_Data.Data_Transfer[16],0,8)BTD(LTF.Write_Data.BDC2_Delay_On_OneShot_Delay,24,Port_Data.Data_Transfer[17],0,8)BTD(LTF.Write_Data.BDC2_Delay_On_OneShot_Delay,16,Port_Data.Data_Transfer[18],0,8)BTD(LTF.Write_Data.BDC2_Delay_On_OneShot_Delay,8,Port_Data.Data_Transfer[19],0,8)BTD(LTF.Write_Data.BDC2_Delay_On_OneShot_Delay,0,Port_Data.Data_Transfer[20],0,8)BTD(LTF.Write_Data.BDC2_Delay_Mode,0,Port_Data.Data_Transfer[21],0,8)MOV(Port,Port_Data.Data_Transfer[185])MOV(0,Port_Data.Data_Transfer[187])MOV(66,Port_Data.Data_Transfer[188])MOV(22,Port_Data.Data_Transfer[189])MOV(9,Inprocess_Index)OTL(Port_Data.Port_Write.[Port])OTL(Local_Control.11);
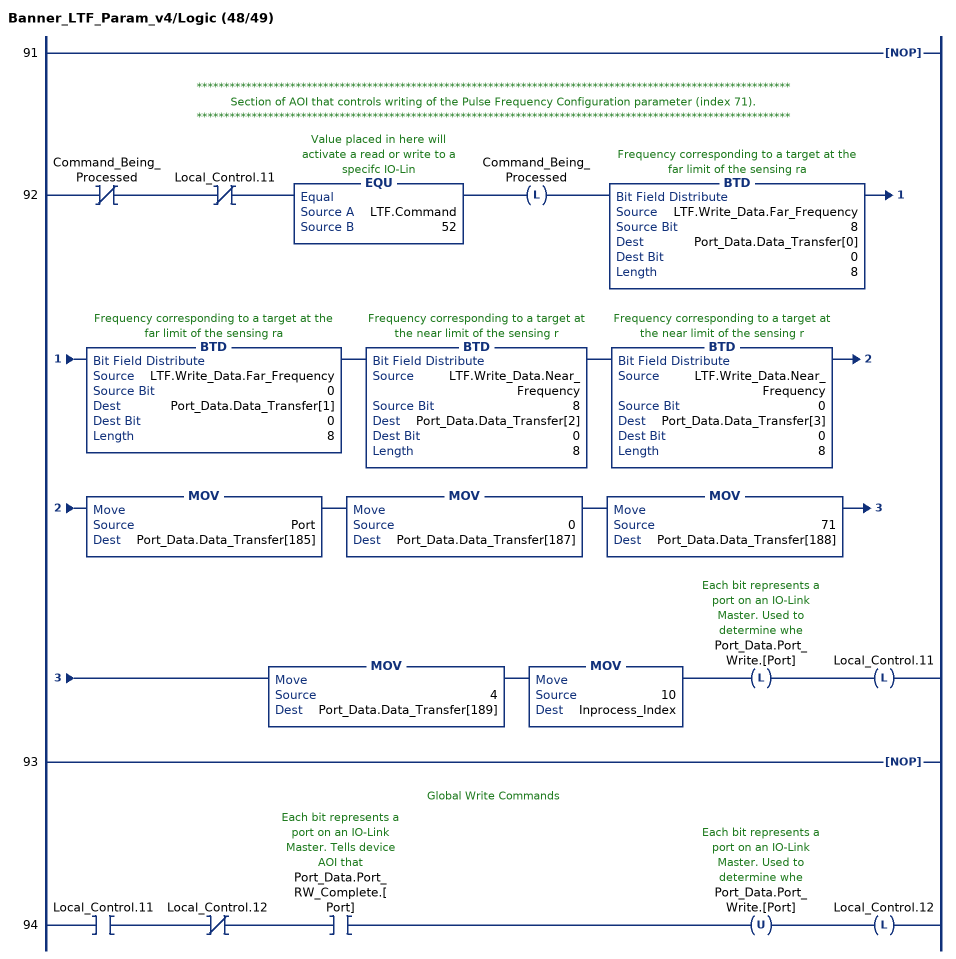
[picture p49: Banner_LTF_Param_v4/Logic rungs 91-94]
   91: NOP();
   // ************************************************************************************************************
   // Section of AOI that controls writing of the Pulse Frequency Configuration parameter (index 71).
   // ************************************************************************************************************
   92: XIO(Command_Being_Processed)XIO(Local_Control.11)EQU(LTF.Command,52)OTL(Command_Being_Processed)BTD(LTF.Write_Data.Far_Frequency,8,Port_Data.Data_Transfer[0],0,8)BTD(LTF.Write_Data.Far_Frequency,0,Port_Data.Data_Transfer[1],0,8)BTD(LTF.Write_Data.Near_Frequency,8,Port_Data.Data_Transfer[2],0,8)BTD(LTF.Write_Data.Near_Frequency,0,Port_Data.Data_Transfer[3],0,8)MOV(Port,Port_Data.Data_Transfer[185])MOV(0,Port_Data.Data_Transfer[187])MOV(71,Port_Data.Data_Transfer[188])MOV(4,Port_Data.Data_Transfer[189])MOV(10,Inprocess_Index)OTL(Port_Data.Port_Write.[Port])OTL(Local_Control.11);
   93: NOP();
   // Global Write Commands
   94: XIC(Local_Control.11)XIO(Local_Control.12)XIC(Port_Data.Port_RW_Complete.[Port])OTU(Port_Data.Port_Write.[Port])OTL(Local_Control.12);
